FUNCTION_BLOCK FB_DO_IED_LD1_LPHD1_PhyNam EXTENDS FB_AcsiCommonDataClass
VAR_INPUT
	vendor: FB_AcsiDATypeVisString255 := (fc:=ACSI_FC_DC, bLinkResult:=THIS^.AddDataToContainer(ipData:=vendor));
	hwRev: FB_AcsiDATypeVisString255 := (fc:=ACSI_FC_DC, bLinkResult:=THIS^.AddDataToContainer(ipData:=hwRev));
	swRev: FB_AcsiDATypeVisString255 := (fc:=ACSI_FC_DC, bLinkResult:=THIS^.AddDataToContainer(ipData:=swRev));
	serNum: FB_AcsiDATypeVisString255 := (fc:=ACSI_FC_DC, bLinkResult:=THIS^.AddDataToContainer(ipData:=serNum));
	model: FB_AcsiDATypeVisString255 := (fc:=ACSI_FC_DC, bLinkResult:=THIS^.AddDataToContainer(ipData:=model));
	location: FB_AcsiDATypeVisString255 := (fc:=ACSI_FC_DC, bLinkResult:=THIS^.AddDataToContainer(ipData:=location));
END_VAR
VAR
END_VAR

END_FUNCTION_BLOCK
